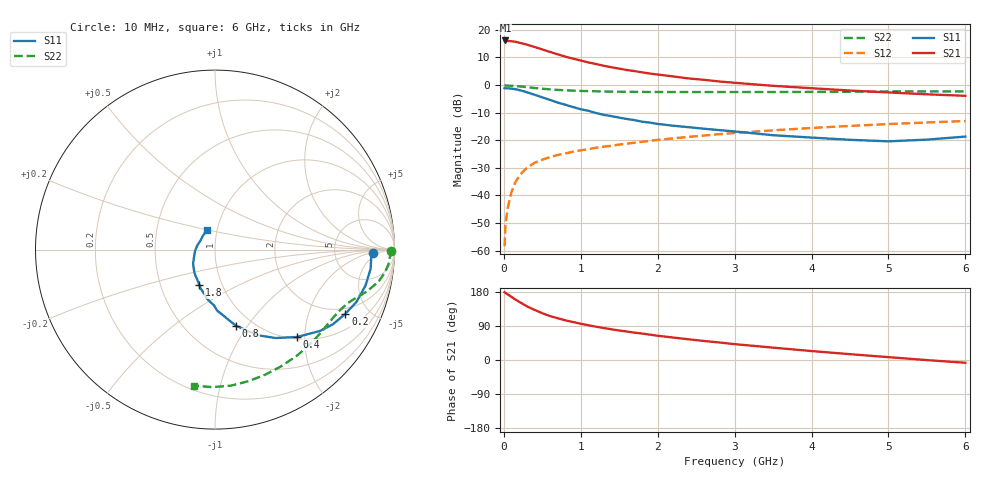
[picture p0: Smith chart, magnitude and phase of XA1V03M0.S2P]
! SIEMENS Discrete & RF Semiconductors
! BFY180
! Si NPN RF Bipolar Junction Transistor in MICRO-X
! VCE = 1 V  IC = 3 mA
! Common Emitter S-Parameters:  May  1997
# GHz  S  MA  R  50
!  f  S11  S21  S12  S22
! GHz  MAG  ANG  MAG  ANG  MAG  ANG  MAG  ANG
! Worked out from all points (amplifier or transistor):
!   36 points, 10 MHz to 6 GHz, reference 50 ohm
!   highest |S21| = 16.2 dB at 20 MHz (marker M1)
!   |S21| within 3 dB of that: start of sweep to 470.9 MHz
!   unconditionally stable (mu >= 1): 869.3 MHz to end of sweep
!   at 250 MHz: K = 0.35, MSG = 23.2 dB, |S12| = -31.3 dB
!   at 1.4 GHz: K = 1.29, MAG = 11.0 dB, |S12| = -22.0 dB
!   at 6 GHz: K = 1.41, MAG = 0.8 dB, |S12| = -13.0 dB
!   S11 on the Smith chart (normalised r, x): 10 MHz: 15, -2; 200 MHz: 1.70, -3.53; 400 MHz: 1.04, -1.83; 800 MHz: 0.84, -0.88; 1.8 GHz: 0.78, -0.32; 6 GHz: 0.89, +0.19
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0.01  0.8781 -1.2  6.306 178.8  0.0012 78.2  0.9789 -0.3
0.02  0.8715 -2.7  6.431 177.1  0.0028 90.5  0.9824 -0.9
0.05  0.8738 -7.0  6.287 173.3  0.0059 83.2  0.9755 -2.4
0.1  0.8622 -13.4  6.225 166.5  0.0116 82.0  0.9704 -4.7
0.15  0.8405 -20.3  6.09 159.7  0.0173 77.5  0.9593 -6.8
0.2  0.8096 -26.2  5.854 153.5  0.0224 74.4  0.9461 -8.8
0.3  0.7397 -37.8  5.409 141.7  0.0315 67.8  0.9141 -12.2
0.4  0.6679 -46.8  4.89 132.1  0.039 62.7  0.8845 -14.8
0.5  0.5978 -55.5  4.421 123.5  0.0444 59.2  0.8574 -16.9
0.6  0.538 -62.8  3.987 115.8  0.0493 56.7  0.8351 -18.5
0.8  0.4388 -74.7  3.269 104.6  0.0575 53.6  0.8023 -21.5
1  0.364 -83.7  2.784 95.7  0.0655 51.6  0.7826 -24.3
1.1  0.3412 -87.8  2.57 91.7  0.0689 51.2  0.7752 -25.6
1.2  0.3105 -91.1  2.4 87.8  0.0731 50.5  0.7701 -27.0
1.4  0.2729 -100.4  2.101 81.0  0.0793 49.7  0.76 -29.8
1.8  0.2164 -113.9  1.697 69.8  0.0937 48.2  0.7509 -35.7
2.2  0.1833 -125.7  1.435 59.3  0.108 46.1  0.7474 -41.8
2.8  0.1524 -142.3  1.16 46.2  0.1288 42.3  0.7462 -50.7
3.5  0.1231 -161.3  0.968 32.6  0.151 37.5  0.7475 -61.0
4.5  0.1017 167.1  0.795 15.4  0.1816 29.6  0.7564 -75.7
5.5  0.1024 131.2  0.679 -0.3  0.2096 21.3  0.7665 -91.2
6  0.1164 113.6  0.638 -7.3  0.2226 16.8  0.7668 -98.9
